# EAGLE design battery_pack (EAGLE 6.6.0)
AUTHOR: Joshua Adkins; REV: A; TITLE: Battery_Pack
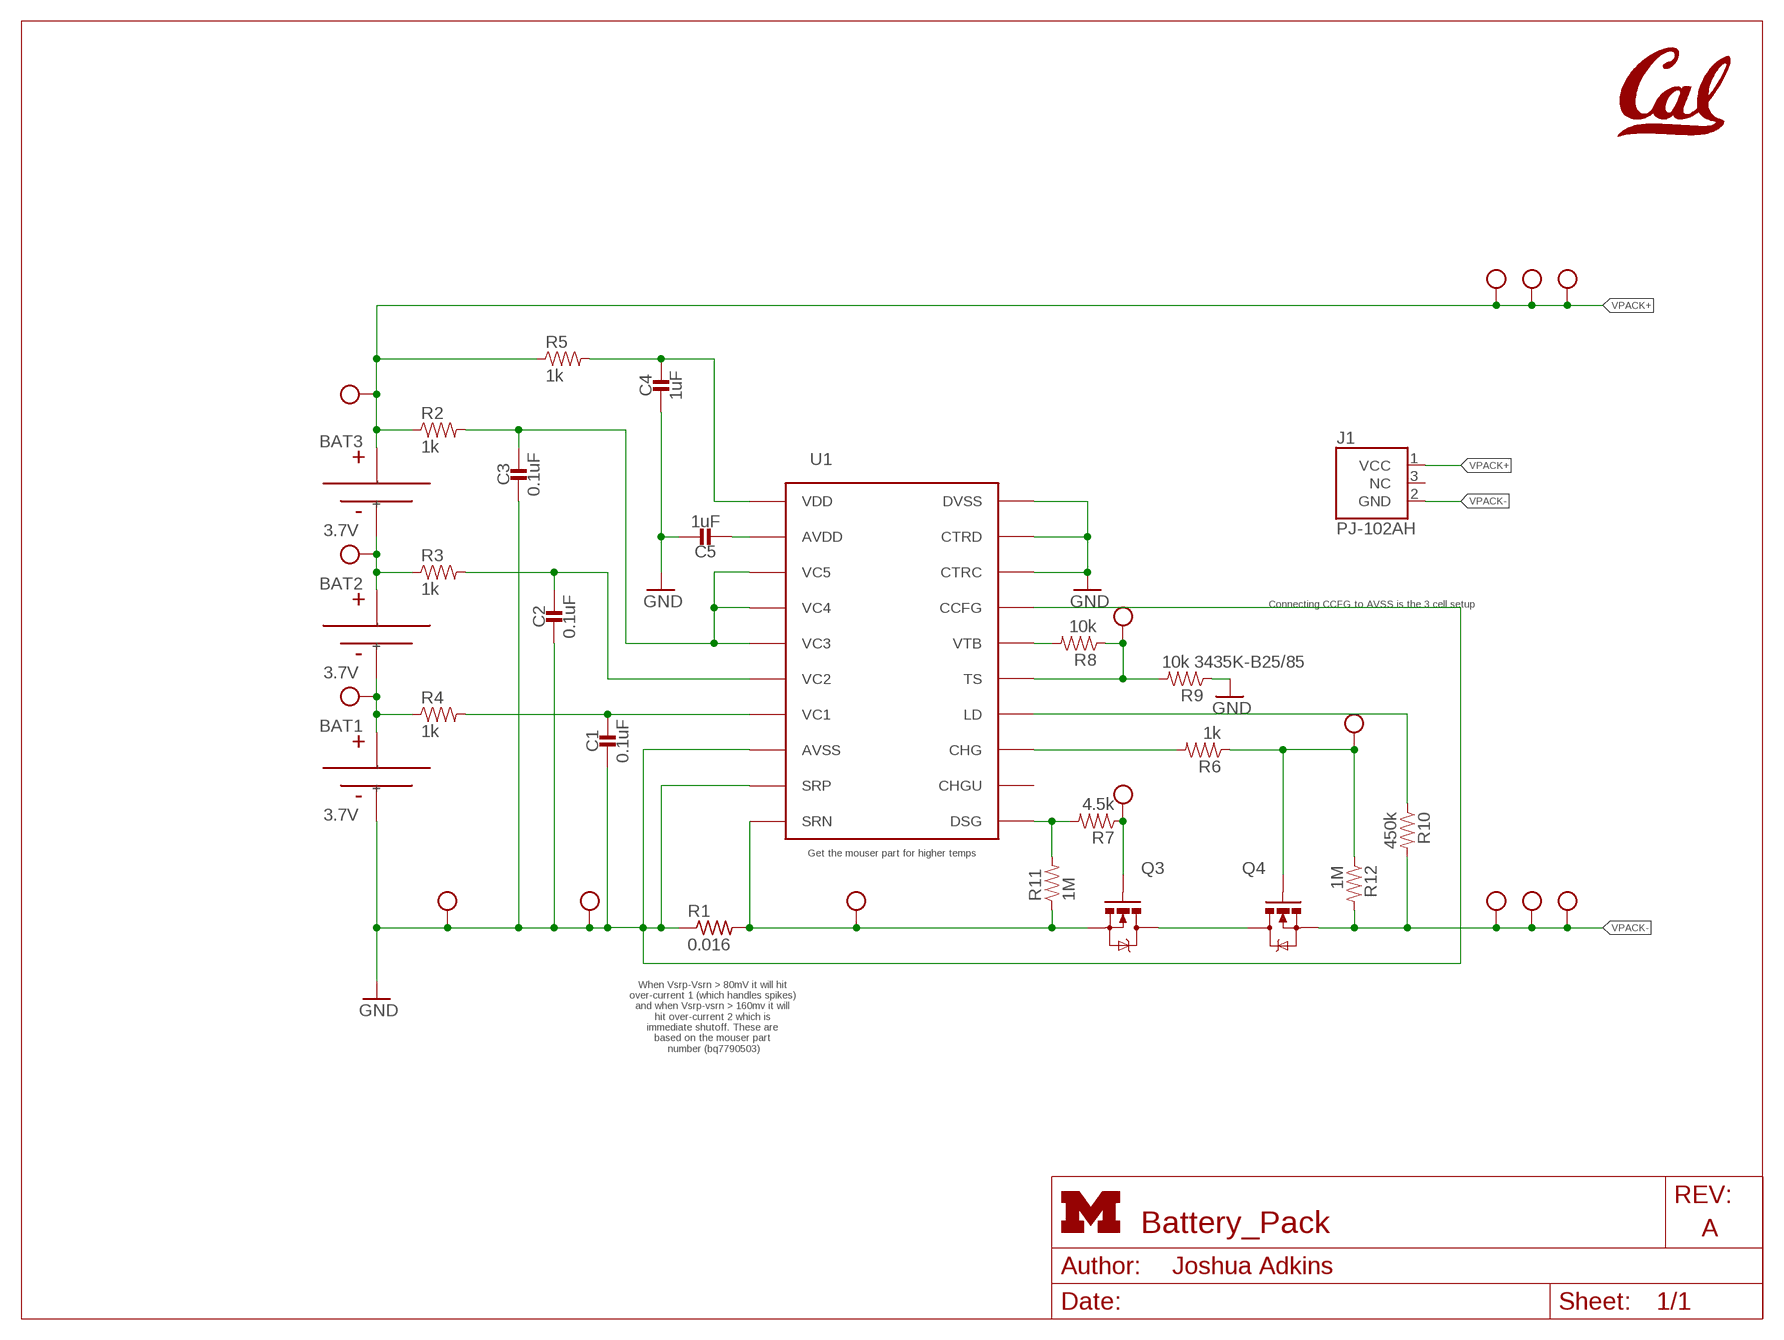
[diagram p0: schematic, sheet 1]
FRAME1 (LETTER_L_UMICH): HEIGHT: 8.5in; WIDTH: 11in

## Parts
BAT1  3.7V  BAT-CELL  [PL-809797-1C]
BAT2  3.7V  BAT-CELL  [PL-809797-1C]
BAT3  3.7V  BAT-CELL  [PL-809797-1C]
C1  0.1uF  CAPACITOR0603_CAP  [0603_CAP]
C2  0.1uF  CAPACITOR0603_CAP  [0603_CAP]
C3  0.1uF  CAPACITOR0603_CAP  [0603_CAP]
C4  1uF  CAPACITOR0603_CAP  [0603_CAP]
C5  1uF  CAPACITOR0603_CAP  [0603_CAP]
J1  PJ-102AH  [PJ-102AH]
Q3  MOSFET-NCHANNELFDD8580  [DPAK]
Q4  MOSFET-NCHANNELFDD8580  [DPAK]
R1  0.016  R-US_R1206  [R1206]
R2  1k  RESISTOR0603_RES  [0603-RES]
R3  1k  RESISTOR0603_RES  [0603-RES]
R4  1k  RESISTOR0603_RES  [0603-RES]
R5  1k  RESISTOR0603_RES  [0603-RES]
R6  1k  RESISTOR0603_RES  [0603-RES]
R7  4.5k  RESISTOR0603_RES  [0603-RES]
R8  10k  RESISTOR0603_RES  [0603-RES]
R9  10k 3435K-B25/85  RESISTOR0603_RES  [0603-RES]
R10  450k  RESISTOR0603_RES  [0603-RES]
R11  1M  RESISTOR0603_RES  [0603-RES]
R12  1M  RESISTOR0603_RES  [0603-RES]
TP1  TEST_POINT_0.112IN  [TESTPOINT_0.112IN]
TP2  TEST_POINT_0.112IN  [TESTPOINT_0.112IN]
TP3  TEST_POINT_0.040IN  [TESTPOINT_0.040IN]
TP4  TEST_POINT_0.040IN  [TESTPOINT_0.040IN]
TP5  TEST_POINT_0.112IN  [TESTPOINT_0.112IN]
TP6  TEST_POINT_0.112IN  [TESTPOINT_0.112IN]
TP7  TEST_POINT_0.112IN  [TESTPOINT_0.112IN]
TP8  TEST_POINT_0.112IN  [TESTPOINT_0.112IN]
TP9  TEST_POINT_0.040IN  [TESTPOINT_0.040IN]
TP10  TEST_POINT_0.040IN  [TESTPOINT_0.040IN]
TP11  TEST_POINT_0.040IN  [TESTPOINT_0.040IN]
TP12  TEST_POINT_0.040IN  [TESTPOINT_0.040IN]
TP13  TEST_POINT_0.040IN  [TESTPOINT_0.040IN]
TP14  TEST_POINT_0.112IN  [TESTPOINT_0.112IN]
TP15  TEST_POINT_0.112IN  [TESTPOINT_0.112IN]
U1  BQ77904  [TSSOP-20/6MM]
U$1  UCB_CAL500MIL  [UCB_CAL_500MIL]

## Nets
GND: BAT1.- C1.2 C2.2 C3.2 C4.2 C5.1 R1.1 R9.1 TP7.1(TESTPOINT) TP9.TESTPOINT U1.8(AVSS) U1.9(SRP) U1.17(CCFG) U1.18(CTRC) U1.19(CTRD) U1.20(DVSS)
N$1: BAT1.+ BAT2.- R4.1 TP15.1(TESTPOINT)
N$2: BAT2.+ BAT3.- R3.1 TP14.1(TESTPOINT)
N$4: C1.1 R4.2 U1.7(VC1)
N$5: C2.1 R3.2 U1.6(VC2)
N$6: C3.1 R2.2 U1.3(VC5) U1.4(VC4) U1.5(VC3)
N$7: Q3.4(D) Q4.4(D)
N$8: Q3.3(S) R1.2 R11.1 TP10.TESTPOINT U1.10(SRN)
N$9: C4.1 R5.2 U1.1(VDD)
N$10: R7.2 R11.2 U1.11(DSG)
N$11: C5.2 U1.2(AVDD)
N$12: Q3.1(G) R7.1 TP11.TESTPOINT
N$13: R6.2 U1.13(CHG)
N$14: Q4.1(G) R6.1 R12.1 TP12.TESTPOINT
N$17: R10.1 U1.14(LD)
N$18: R8.2 U1.16(VTB)
N$19: R8.1 R9.2 TP13.TESTPOINT U1.15(TS)
VPACK+: BAT3.+ J1.1(VCC) R2.1 R5.1 TP1.1(TESTPOINT) TP3.TESTPOINT TP6.1(TESTPOINT) TP8.1(TESTPOINT)
VPACK-: J1.2(GND) Q4.3(S) R10.2 R12.2 TP2.1(TESTPOINT) TP4.TESTPOINT TP5.1(TESTPOINT)
Unconnected: J1.3(NC) U1.12(CHGU)

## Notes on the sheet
- Connecting CCFG to AVSS is the 3 cell setup
- Get the mouser part for higher temps
- When Vsrp-Vsrn > 80mV it will hit 
  over-current 1 (which handles spikes) 
  and when Vsrp-vsrn > 160mv it will 
  hit over-current 2 which is 
  immediate shutoff. These are 
  based on the mouser part 
  number (bq7790503)

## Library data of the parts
BAT1-BAT3 = batteries:BAT-CELL: A single cell of a battery
C1-C5 = passives:CAPACITOR: 0402 Capacitor
J1 = connector:PJ-102AH: DC Power Jack 2.0mm / 5.5mm; DIGIKEY: CP-102AH-ND
Q3 Q4 = fets:MOSFET-NCHANNEL: Generic NMOS footprint
R1 = resistor:R-US_: RESISTOR, American symbol
R2-R12 = passives:RESISTOR: Resistor
TP1 TP2 TP5-TP8 TP14 TP15 = headers:TEST_POINT_0.112IN: Solder terminal, turreted; NEWARK: 40F6015
TP3 TP4 TP9-TP13 = headers:TEST_POINT_0.040IN: 0.040in Test Point; DIGIKEY: 5001K-ND
U1 = chips:BQ77904: A battery protection chip with OV/UV/OT/UT; DIGIKEY: 296-44599-5-ND; MOUSER: 595-BQ7790503PW
U$1 = logos:UCB_CAL

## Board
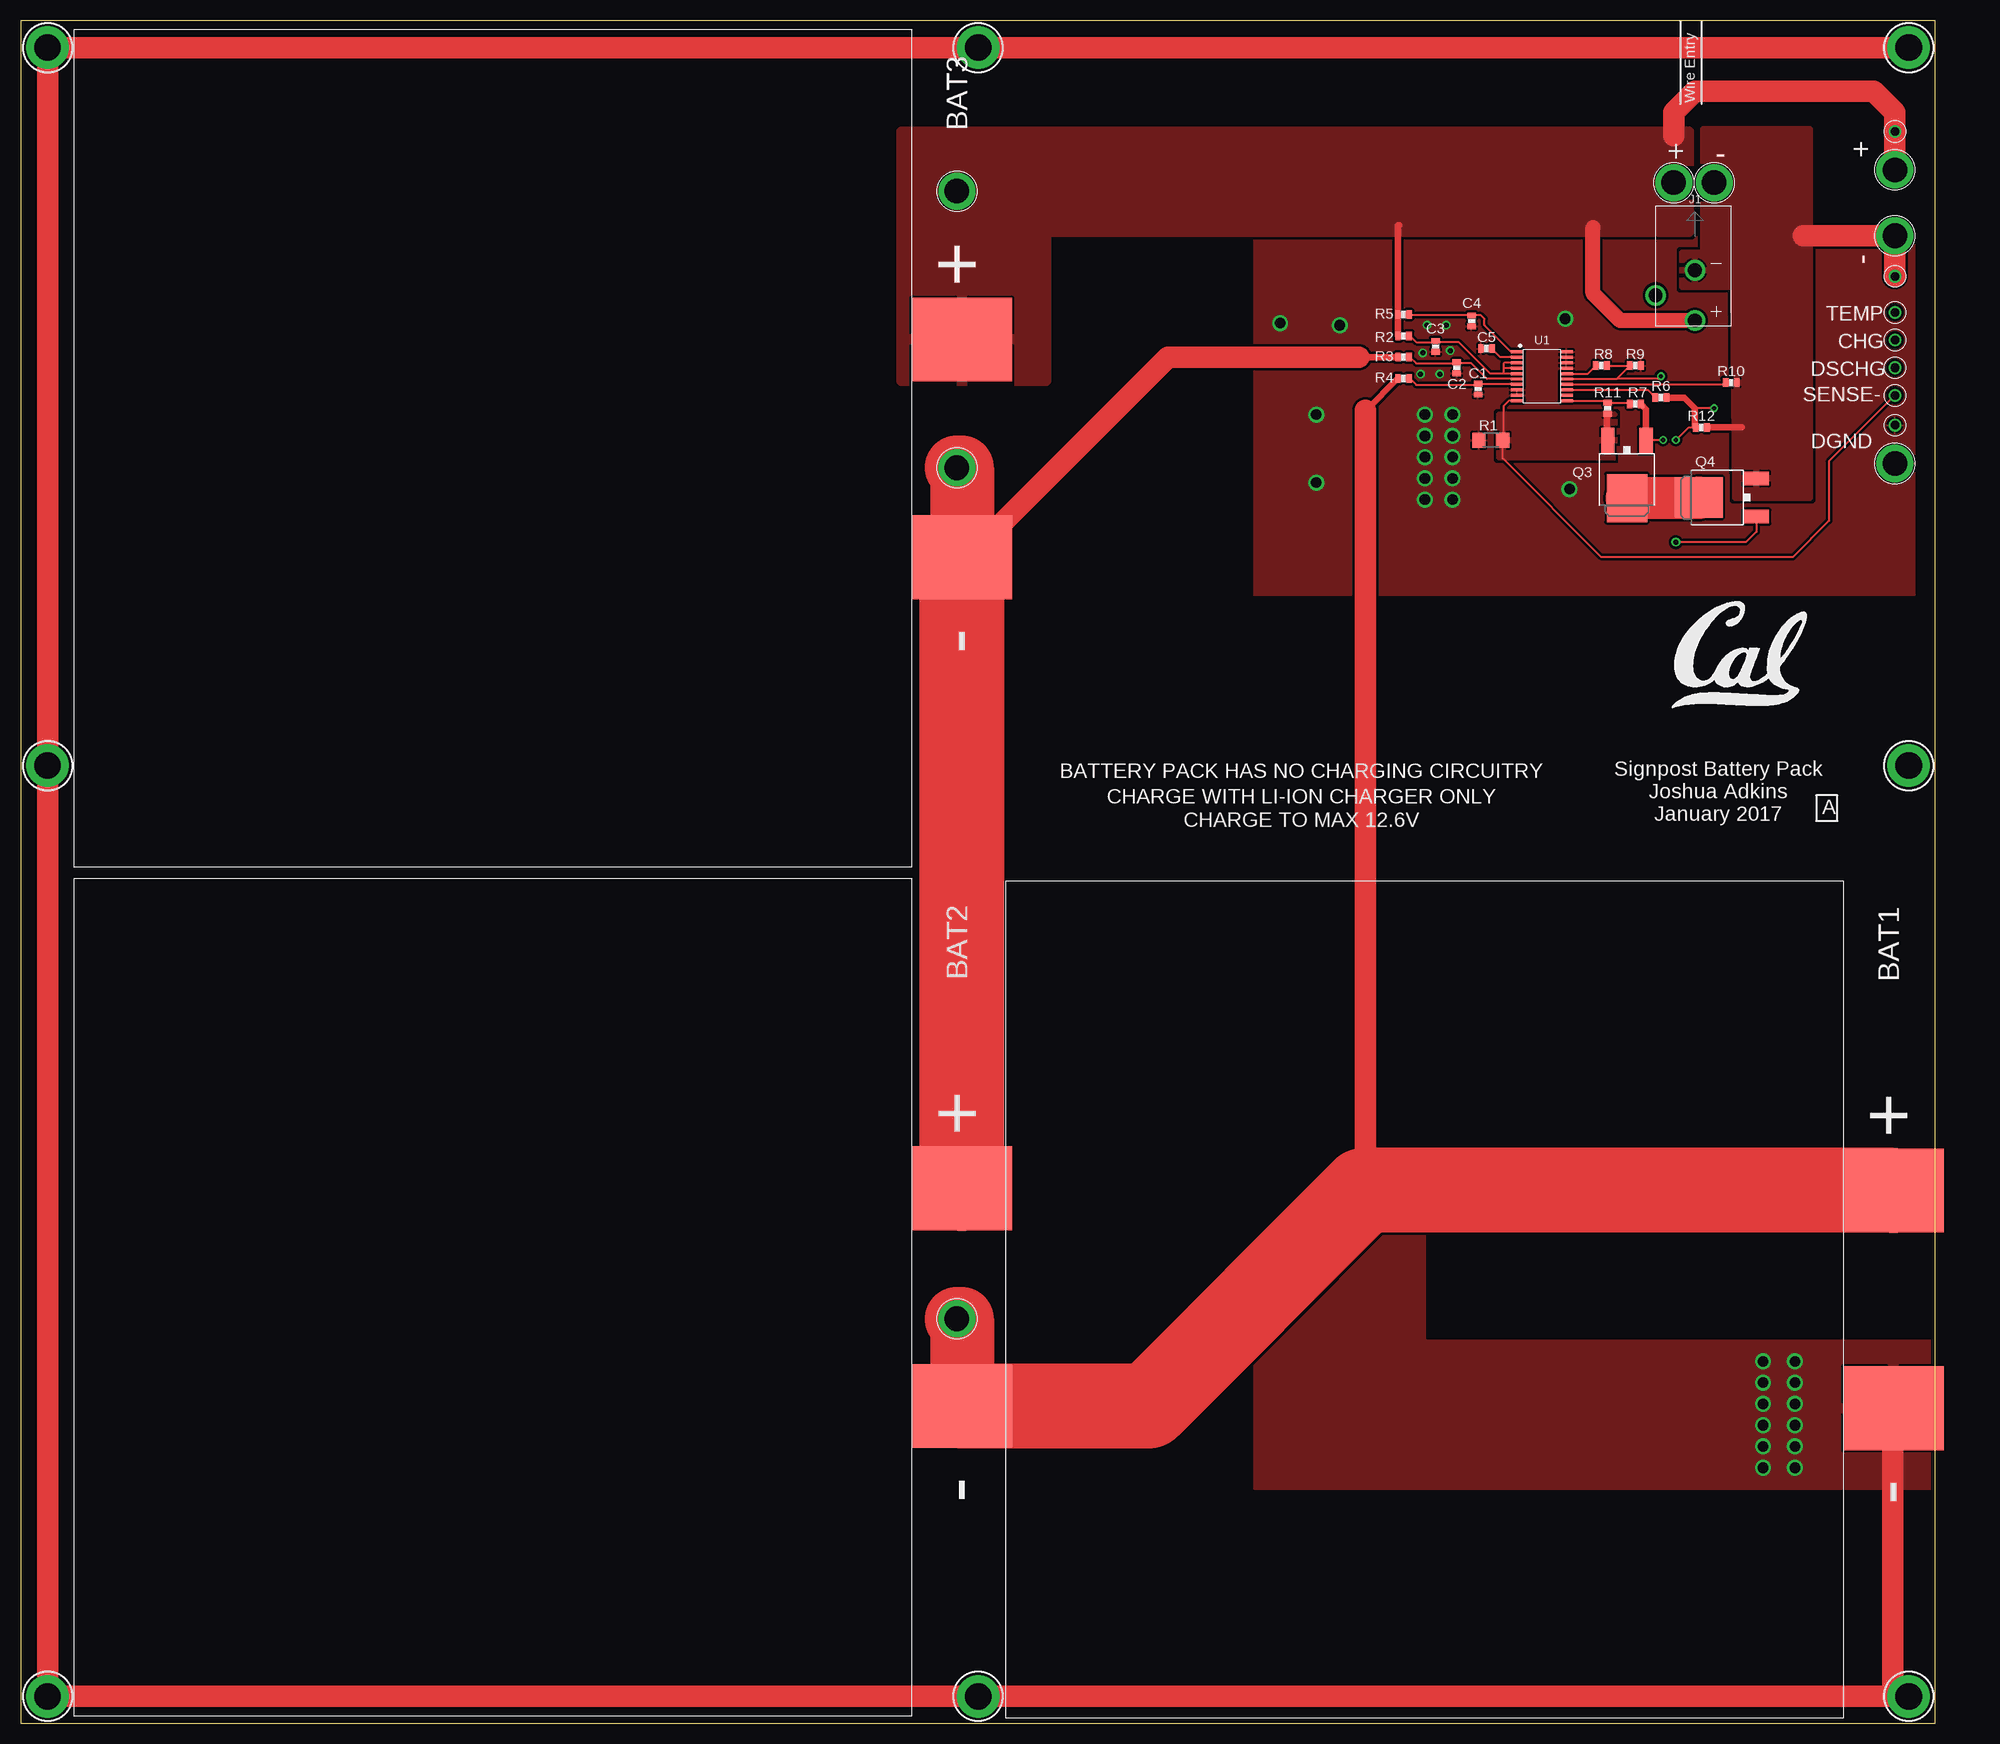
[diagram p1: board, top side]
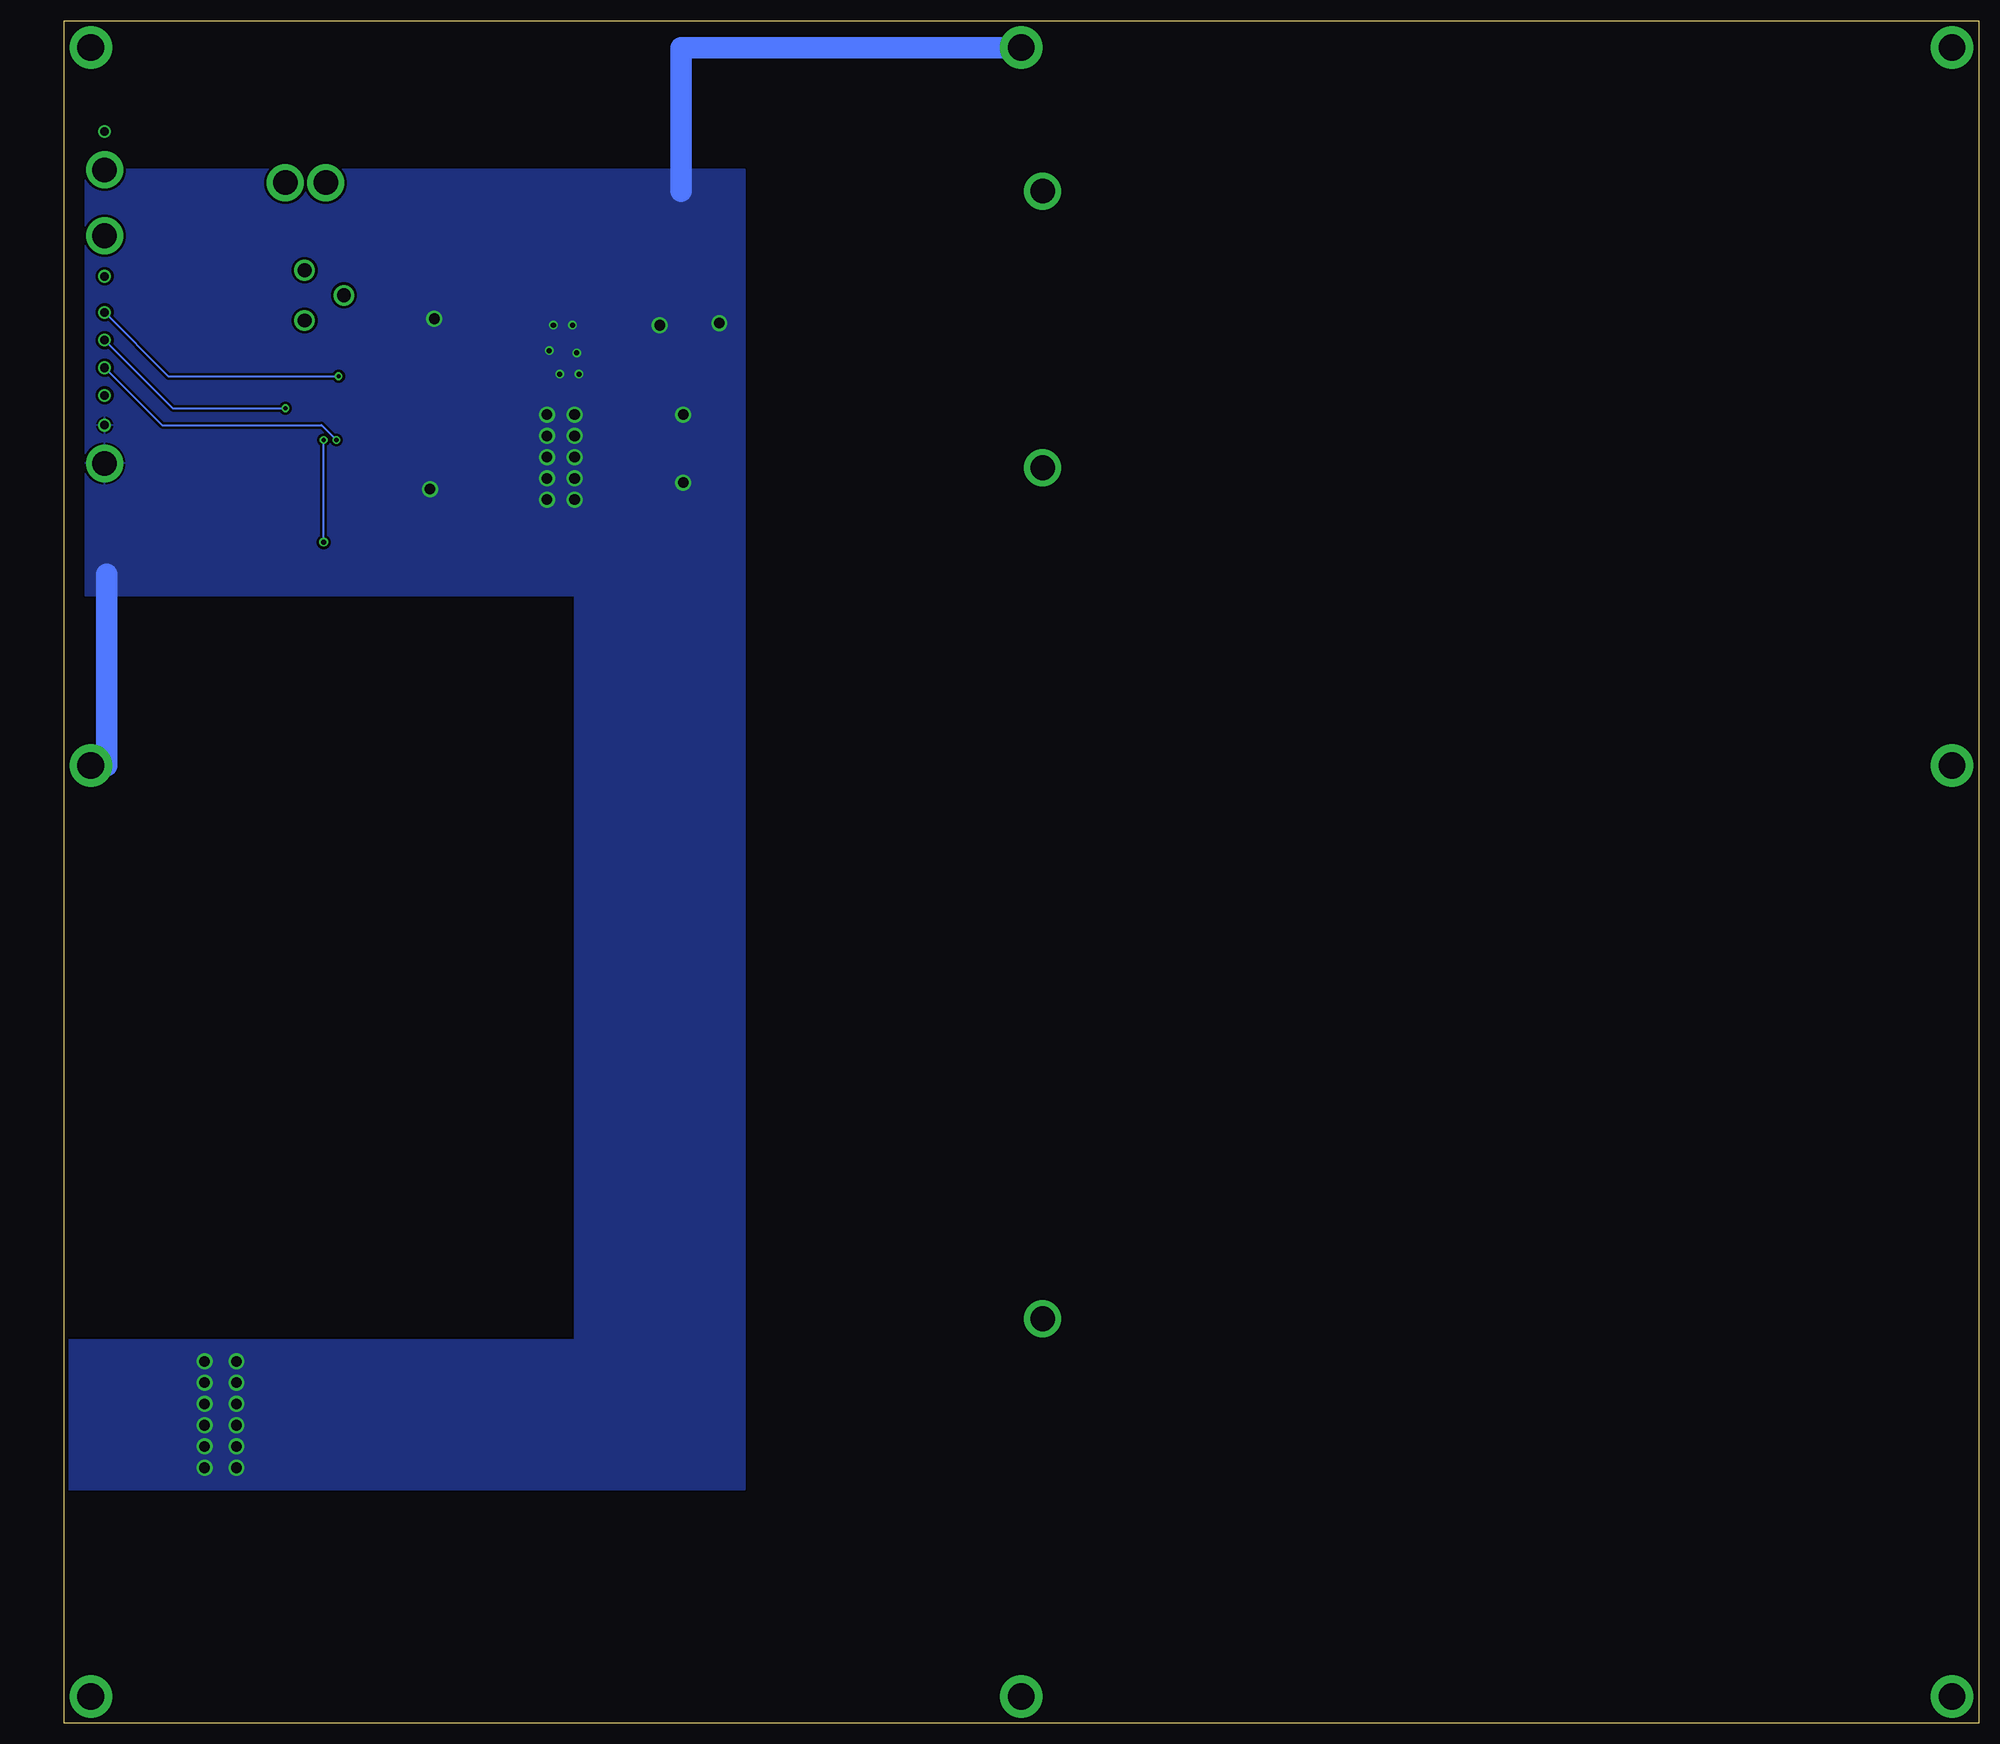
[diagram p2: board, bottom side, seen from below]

Size 228.6 x 203.2 mm. Coordinates in mm from the lower left corner, seen from the top.
Outline: 0,0 228.58,0 228.6,203.2 0,203.2 0,0
Copper layers (1*16): Top 0.0178mm / dielectric 59mil / Bottom 0.0178mm
Design rules "quickturn_co_kr_1oz": minimum track width 4mil, minimum drill 0.200659375mm, track to track 4mil, track to pad 4mil, pad to pad 4mil, via to via 4mil, smd to smd 4mil, copper to edge 20mil, drill to drill 16mil, minimum pad ring 8mil, minimum via ring 8mil, stop-mask expansion 3mil, vias tented up to drill 50mil, thermal gap 10mil

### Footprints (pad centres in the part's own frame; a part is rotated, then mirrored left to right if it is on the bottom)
PL-809797-1C = smd 10 x 12: + 37,106; - 63,106
0603_CAP = smd 0.7 x 1: 1 -0.65,0; 2 0.65,0
PJ-102AH = drill 1.65: 1 0,-3; 2 0,3; 3 -4.7,0
DPAK = smd 1.6 x 3: 1 -2.28,-5.31; 3 2.28,-5.31 | smd 4.826 x 5.715: 4 0,1.588
R1206 = smd 1.6 x 1.803: 1 -1.422,0; 2 1.422,0
0603-RES = smd 0.7 x 1: 1 -0.65,0; 2 0.65,0
TESTPOINT_0.112IN = drill 2.946: 1 0,0
TESTPOINT_0.040IN = drill 1.016: TESTPOINT 0,0
TSSOP-20/6MM = smd 1.5 x 0.35: 1 -2.95,2.925; 2 -2.95,2.275; 3 -2.95,1.625; 4 -2.95,0.975; 5 -2.95,0.325; 6 -2.95,-0.325; 7 -2.95,-0.975; 8 -2.95,-1.625; 9 -2.95,-2.275; 10 -2.95,-2.925; 11 2.95,-2.925; 12 2.95,-2.275; 13 2.95,-1.625; 14 2.95,-0.975; 15 2.95,-0.325; 16 2.95,0.325; 17 2.95,0.975; 18 2.95,1.625; 19 2.95,2.275; 20 2.95,2.925

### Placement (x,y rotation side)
BAT1  117.6,100.58 270 top
BAT2  6.35,100.84 270 top
BAT3  6.35,202.18 270 top
C1  173.99,159.26 270 top
C2  171.45,161.8 270 top
C3  168.91,164.34 270 top
C4  173.23,167.39 270 top
C5  175.01,164.08 0 top
J1  199.9,170.43 0 top
Q3  191.77,147.83 180 top
Q4  201.93,146.3 90 top
R1  175.51,153.16 0 top
R2  165.1,165.61 0 top
R3  165.1,163.07 0 top
R4  165.1,160.53 0 top
R5  165.1,168.15 0 top
R6  195.83,158.24 180 top
R7  192.79,157.48 180 top
R8  188.72,162.05 180 top
R9  192.79,162.05 180 top
R10  204.22,160.02 0 top
R11  189.48,156.97 90 top
R12  200.66,154.69 0 top
TP1  197.36,183.9 0 top
TP2  223.77,177.55 0 top
TP3  223.77,189.99 0 top
TP4  223.77,172.72 0 top
TP5  202.18,183.9 0 top
TP6  223.77,185.42 0 top
TP7  223.77,150.37 0 top
TP8  111.76,182.88 0 top
TP9  223.77,154.94 0 top
TP10  223.77,158.5 90 top
TP11  223.77,161.8 90 top
TP12  223.77,165.1 90 top
TP13  223.77,168.4 90 top
TP14  111.76,149.86 0 top
TP15  111.76,48.26 0 top
U1  181.61,160.78 0 top
U$1  197.1,121.16 0 top

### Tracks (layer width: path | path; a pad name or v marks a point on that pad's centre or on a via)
GND  (via drill 0.61, 1.27, 3.17 pad 5.08)
  Top 2.54: 223.52,38.1 223.52,3.17 v225.43,3.17 v114.3,3.17 v3.17,3.17 v3.17,114.3 | v3.17,114.3 v3.17,200.03 v114.3,200.03 v225.43,200.03 | v3.17,114.3 2.54,114.3
  Bottom 2.54: v114.3,200.03 154.94,200.03 154.94,182.88 | v225.43,114.3 223.52,114.3 223.52,137.16
  other vias: 167.89,166.88 170.18,166.88 167.39,163.58 167.13,161.04 169.42,161.04 170.69,163.83 157.48,166.88 167.64,153.67 167.64,146.05 184.91,147.32 184.4,167.64 150.37,167.13 154.69,156.21 154.69,148.08 211.84,43.18 211.84,40.64 211.84,38.1 211.84,35.56 211.84,33.02 211.84,30.48 208.03,43.18 208.03,40.64 208.03,38.1 208.03,35.56 208.03,33.02 208.03,30.48 167.64,148.59 167.64,151.13 167.64,156.21 170.94,146.05 170.94,148.59 170.94,151.13 170.94,153.67 170.94,156.21
  pour Bottom (isolate 0.305): 147.32,185.42 226.06,185.42 226.06,134.62 147.32,134.62
  pour Top (isolate 0.305, rank 2): 147.32,185.42 226.06,185.42 226.06,134.62 147.32,134.62
  pour Top (isolate 0.305): 216.41,43.94 216.41,29.97 228.35,29.97 228.35,43.94
  pour Bottom (isolate 0.305): 228.6,27.94 147.32,27.94 147.32,144.78 167.64,144.78 167.64,45.72 228.6,45.72
  pour Top (isolate 0.305): 228.6,27.94 147.32,27.94 147.32,144.78 167.64,144.78 167.64,45.72 228.6,45.72
N$1
  Top 0.254: 160.53,156.72 160.64,156.72
  Top 0.762: 160.64,156.72 R4.1
  Top 10.16: BAT1.+ 160.36,63.58 159.89,63.12 134.62,37.85 BAT2.-
  Top 2.54: 160.53,156.72 160.53,63.75 159.89,63.12
  Top 7.62: TP15.1 112.35,48.26 BAT2.-
N$2
  Top 0.762: R3.1 159.77,163.07
  Top 10.16: BAT2.+ 112.35,137.16 112.35,138.43 BAT3.-
  Top 2.54: 159.77,163.07 136.99,163.07 112.35,138.43
  Top 7.62: TP14.1 112.35,149.86 112.35,137.16
N$4
  Top 0.254: R4.2 165.86,160.53 166.62,159.77 173.85,159.77 C1.1 174.09,159.81 U1.7
N$5
  Top 0.254: U1.6 175.08,160.46 173.23,162.31 171.59,162.31 C2.1 171.31,162.31 166.62,162.31 165.86,163.07 R3.2
N$6
  Top 0.254: U1.5 177.04,161.11 | 177.04,161.11 175.44,161.11 171.7,164.85 169.05,164.85 C3.1 168.77,164.85 166.62,164.85 165.86,165.61 R2.2 | U1.3 177.14,162.41 177.04,162.31 177.04,161.8 | 177.04,161.8 177.04,161.11 | U1.4 177.08,161.76 177.04,161.8
N$7
  Top 5.08: Q3.4 Q4.4
N$8
  Top 0.254: U1.10 177.67,157.86 177.04,157.23 177.04,153.26 R1.2 176.94,150.98 188.72,139.19 211.58,139.19 215.9,143.51 215.9,150.62 TP10.TESTPOINT
  Top 0.762: 189.36,153.26 189.36,156.2 R11.1
  Top 1.27: 189.36,153.26 Q3.3
  pour Top (isolate 0.305): 176.53,151.13 190.25,151.13 190.25,156.21 176.53,156.21
N$9
  Top 0.254: R5.2 173.12,168.15 C4.1 174.36,168.04 174.75,167.64 174.75,166.88 177.92,163.71 U1.1
N$10
  Top 0.254: U1.11 189.25,157.86 R11.2 191.99,157.62 R7.2
N$11
  Top 0.254: U1.2 176.68,163.06 C5.2
N$12  (via drill 0.51)
  Top 0.254: v196.09,153.16 194.07,153.16 Q3.1
  Top 0.762: Q3.1 194.05,156.87 R7.1
  Bottom 0.254: TP11.TESTPOINT 216.92,154.94 197.87,154.94 v196.09,153.16
N$13
  Top 0.254: U1.13 194.27,159.16 R6.2
N$14  (via drill 0.51, 0.61)
  Top 0.254: Q4.1 207.24,142.22 205.99,140.97 v197.61,140.97 | v197.61,153.16 199.14,154.69 R12.1 199.9,154.8 | v202.18,156.97 199.9,156.97
  Top 0.762: R6.1 198.63,158.24 199.9,156.97 199.9,154.8
  Bottom 0.254: v197.61,140.97 v197.61,153.16 | TP12.TESTPOINT 215.65,156.97 v202.18,156.97
N$17
  Top 0.254: U1.14 203.35,159.81 R10.1
N$18
  Top 0.254: U1.16 187.13,161.11 R8.2
N$19  (via drill 0.51)
  Top 0.254: R8.1 R9.2 190.54,160.46 | U1.15 190.54,160.46 | v195.83,160.78 195.51,160.46 190.54,160.46
  Bottom 0.254: TP13.TESTPOINT 216.15,160.78 v195.83,160.78
VPACK+
  Top 0.762: R2.1 R5.1 164.45,178.82 164.59,178.82
  Top 1.778: J1.1 190.96,167.43 187.71,170.69 187.71,178.56
  Top 2.54: TP6.1 TP3.TESTPOINT 223.77,192.28 221.23,194.82 199.9,194.82 197.36,192.28 197.36,189.48
  pour Top (isolate 0.305): 105.16,160.27 105.16,189.99 199.14,189.99 199.14,178.05 122.43,178.05 122.43,160.53 122.43,160.27
VPACK-
  Top 0.762: R12.2 205.49,154.69
  Top 2.54: 212.85,177.55 TP2.1 TP4.TESTPOINT
  pour Top (isolate 0.305): 204.72,146.3 204.47,171.45 198.37,171.45 198.37,175.51 200.91,175.51 200.91,190.25 213.61,190.25 213.61,146.3

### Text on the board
tPlace: Wire Entry | - | + | + | - | TEMP | CHG | DSCHG | SENSE- | DGND | BATTERY PACK HAS NO CHARGING CIRCUITRY | CHARGE WITH LI-ION CHARGER ONLY | Signpost Battery Pack / Joshua Adkins / January 2017 | A | CHARGE TO MAX 12.6V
